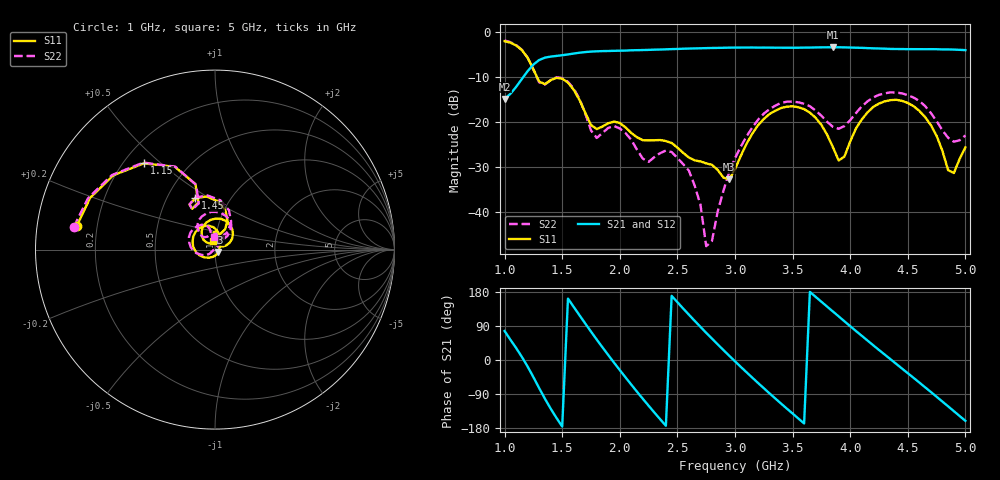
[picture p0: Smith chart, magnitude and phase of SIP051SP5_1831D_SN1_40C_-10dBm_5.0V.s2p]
# GHz  S  dB  R  50
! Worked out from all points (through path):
!   81 points, 1 GHz to 5 GHz, reference 50 ohm
!   highest |S21| = -3.49 dB at 3.85 GHz (marker M1); lowest = -14.9 dB at 1 GHz (marker M2)
!   lowest |S11| = -32.9 dB at 2.95 GHz (marker M3), VSWR 1.05, Z = 51.8 - j1.42 ohm
!   |S11| at or under -10 dB: 1.28 GHz to end of sweep
!   |S22| runs from -47.7 to -2.0 dB; largest |S21 - S12| = 0.0031
!   S11 on the Smith chart (normalised r, x): 1 GHz: 0.12, +0.08; 1.15 GHz: 0.28, +0.44; 1.45 GHz: 0.69, +0.43; 5 GHz: 0.97, +0.10
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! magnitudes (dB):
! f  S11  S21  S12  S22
! 1 GHz  -2.1  -14.9  -15.0  -2.0
! 1.15 GHz  -4.1  -10.5  -10.5  -4.0
! 1.3 GHz  -11.1  -6.3  -6.3  -11.3
! 1.45 GHz  -10.3  -5.4  -5.4  -10.2
! 1.7 GHz  -18.0  -4.6  -4.6  -18.2
! 1.8 GHz  -21.7  -4.4  -4.4  -23.6
! 1.95 GHz  -20.0  -4.3  -4.3  -21.0
! 2.35 GHz  -24.1  -4.0  -4.0  -27.0
! 2.6 GHz  -28.0  -3.8  -3.8  -30.9
! 2.7 GHz  -28.8  -3.7  -3.7  -38.4
! 2.75 GHz  -29.3  -3.7  -3.7  -47.7
! 2.95 GHz  -32.9  -3.6  -3.6  -31.2
! 3 GHz  -30.6  -3.6  -3.6  -28.1
! 3.3 GHz  -18.3  -3.6  -3.6  -17.3
! 3.7 GHz  -19.2  -3.5  -3.5  -17.6
! 3.85 GHz  -25.7  -3.5  -3.5  -21.2
! 3.95 GHz  -27.8  -3.5  -3.5  -21.0
! 4.15 GHz  -18.0  -3.7  -3.7  -15.5
! 4.35 GHz  -15.2  -3.9  -3.8  -13.5
! 4.65 GHz  -19.0  -3.9  -3.9  -16.6
! 4.85 GHz  -30.8  -4.0  -4.0  -23.6
! 5 GHz  -25.7  -4.1  -4.1  -23.1
